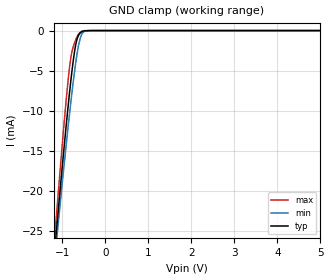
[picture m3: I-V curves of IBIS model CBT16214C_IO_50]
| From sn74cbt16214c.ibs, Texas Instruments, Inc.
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[Model]   CBT16214C_IO_50
Model_type  Terminator
| variable   typ   min   max
C_comp   8.88pF   7.23pF   13.48pF
| C_tri-state   8.88pF   7.23pF   13.48pF
[Temperature Range]   40   100   -40
| Ambient temperature   25   85   -40
[Voltage range]   5   4.5   5.5
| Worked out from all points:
|   GND clamp passes 1 mA (typ) near -0.65 V on its own axis
[GND Clamp]
| CBT16214C_IO_50
|   Voltage   I(typ)   I(min)   I(max)
-5V       -286.8mA   -267.4mA   -310.4mA
-1.155V   -26.34mA   -27.63mA   -24.6mA
-1.12V    -24.23mA   -25.7mA    -22.25mA
-1.085V   -22.14mA   -23.78mA   -19.92mA
-925mV    -12.91mA   -15.25mA   -9.772mA
-815mV    -7.098mA   -9.758mA   -4.034mA
-760mV    -4.527mA   -7.197mA   -2.369mA
-680mV    -1.666mA   -3.863mA   -1.08mA
-610mV    -508.1uA   -1.615mA   -384.4uA
-545mV    -149.1uA   -475uA     -90.52uA
-315mV    -1.002uA   -5.13uA    -27.46nA
5V        831.3pA    2.243nA    368.2pA
